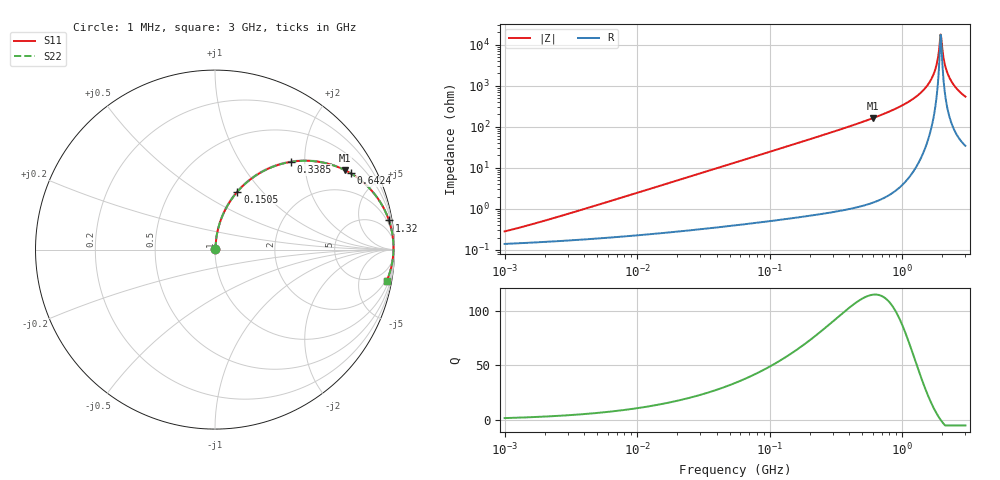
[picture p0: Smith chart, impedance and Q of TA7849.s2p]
# MHz S MA R 50
!Freq  MagS11  AngS11  MagS21  AngS21  MagS12  AngS12  MagS22  AngS22
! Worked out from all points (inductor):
!   801 points, 1 MHz to 3 GHz, reference 50 ohm
!   read as one part in series: L = 39 nH near 1.917 MHz
!   highest Q = 115 at 598.9 MHz (marker M1), where L = 43 nH
!   self-resonance near 1.951 GHz
!   S11 on the Smith chart (normalised r, x): 1 MHz: 1.00, +0.00; 150.5 MHz: 1.01, +0.74; 338.5 MHz: 1.02, +1.71; 642.4 MHz: 1.03, +3.53; 1.32 GHz: 1, +12; 3 GHz: 2, -11
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1  0.002818 60.1  0.9986 -0.1  0.9986 -0.1  0.002818 60.1
3.823119  0.009519 78.7  0.9982 -0.5  0.9982 -0.5  0.009519 78.7
14.47069  0.03544 83.9  0.9969 -2.0  0.9969 -2.0  0.03544 83.9
54.77226  0.1327 80.7  0.9873 -7.6  0.9873 -7.6  0.1327 80.7
150.5037  0.3461 68.8  0.9327 -20.2  0.9327 -20.2  0.3461 68.8
209.4008  0.4582 62.0  0.8827 -27.3  0.8827 -27.3  0.4582 62.0
338.5367  0.6466 49.1  0.7561 -40.3  0.7561 -40.3  0.6466 49.1
598.8949  0.8476 31.6  0.5233 -57.9  0.5233 -57.9  0.8476 31.6
642.3554  0.8668 29.4  0.4912 -60.1  0.4912 -60.1  0.8668 29.4
792.5923  0.9155 23.2  0.3939 -66.3  0.3939 -66.3  0.9155 23.2
1059.487  0.9619 15.2  0.2617 -74.1  0.2617 -74.1  0.9619 15.2
1320.433  0.9827 9.5  0.1652 -79.3  0.1652 -79.3  0.9827 9.5
1534.307  0.9908 5.8  0.1013 -81.9  0.1013 -81.9  0.9908 5.8
1695.807  0.9937 3.4  0.05938 -82.2  0.05938 -82.2  0.9937 3.4
1782.824  0.9944 2.2  0.03864 -80.6  0.03864 -80.6  0.9944 2.2
1893.158  0.9946 0.8  0.01437 -67.7  0.01437 -67.7  0.9946 0.8
1950.859  0.9945 0.1  0.00559 -9.3  0.00559 -9.3  0.9945 0.1
2010.32  0.9942 -0.7  0.01291 62.8  0.01291 62.8  0.9942 -0.7
2134.733  0.993 -2.1  0.037 78.0  0.037 78.0  0.993 -2.1
2289.646  0.9907 -3.8  0.06593 80.0  0.06593 80.0  0.9907 -3.8
2581.816  0.9845 -6.6  0.116 79.0  0.116 79.0  0.9845 -6.6
3000  0.9725 -10.3  0.1793 76.0  0.1793 76.0  0.9725 -10.3
